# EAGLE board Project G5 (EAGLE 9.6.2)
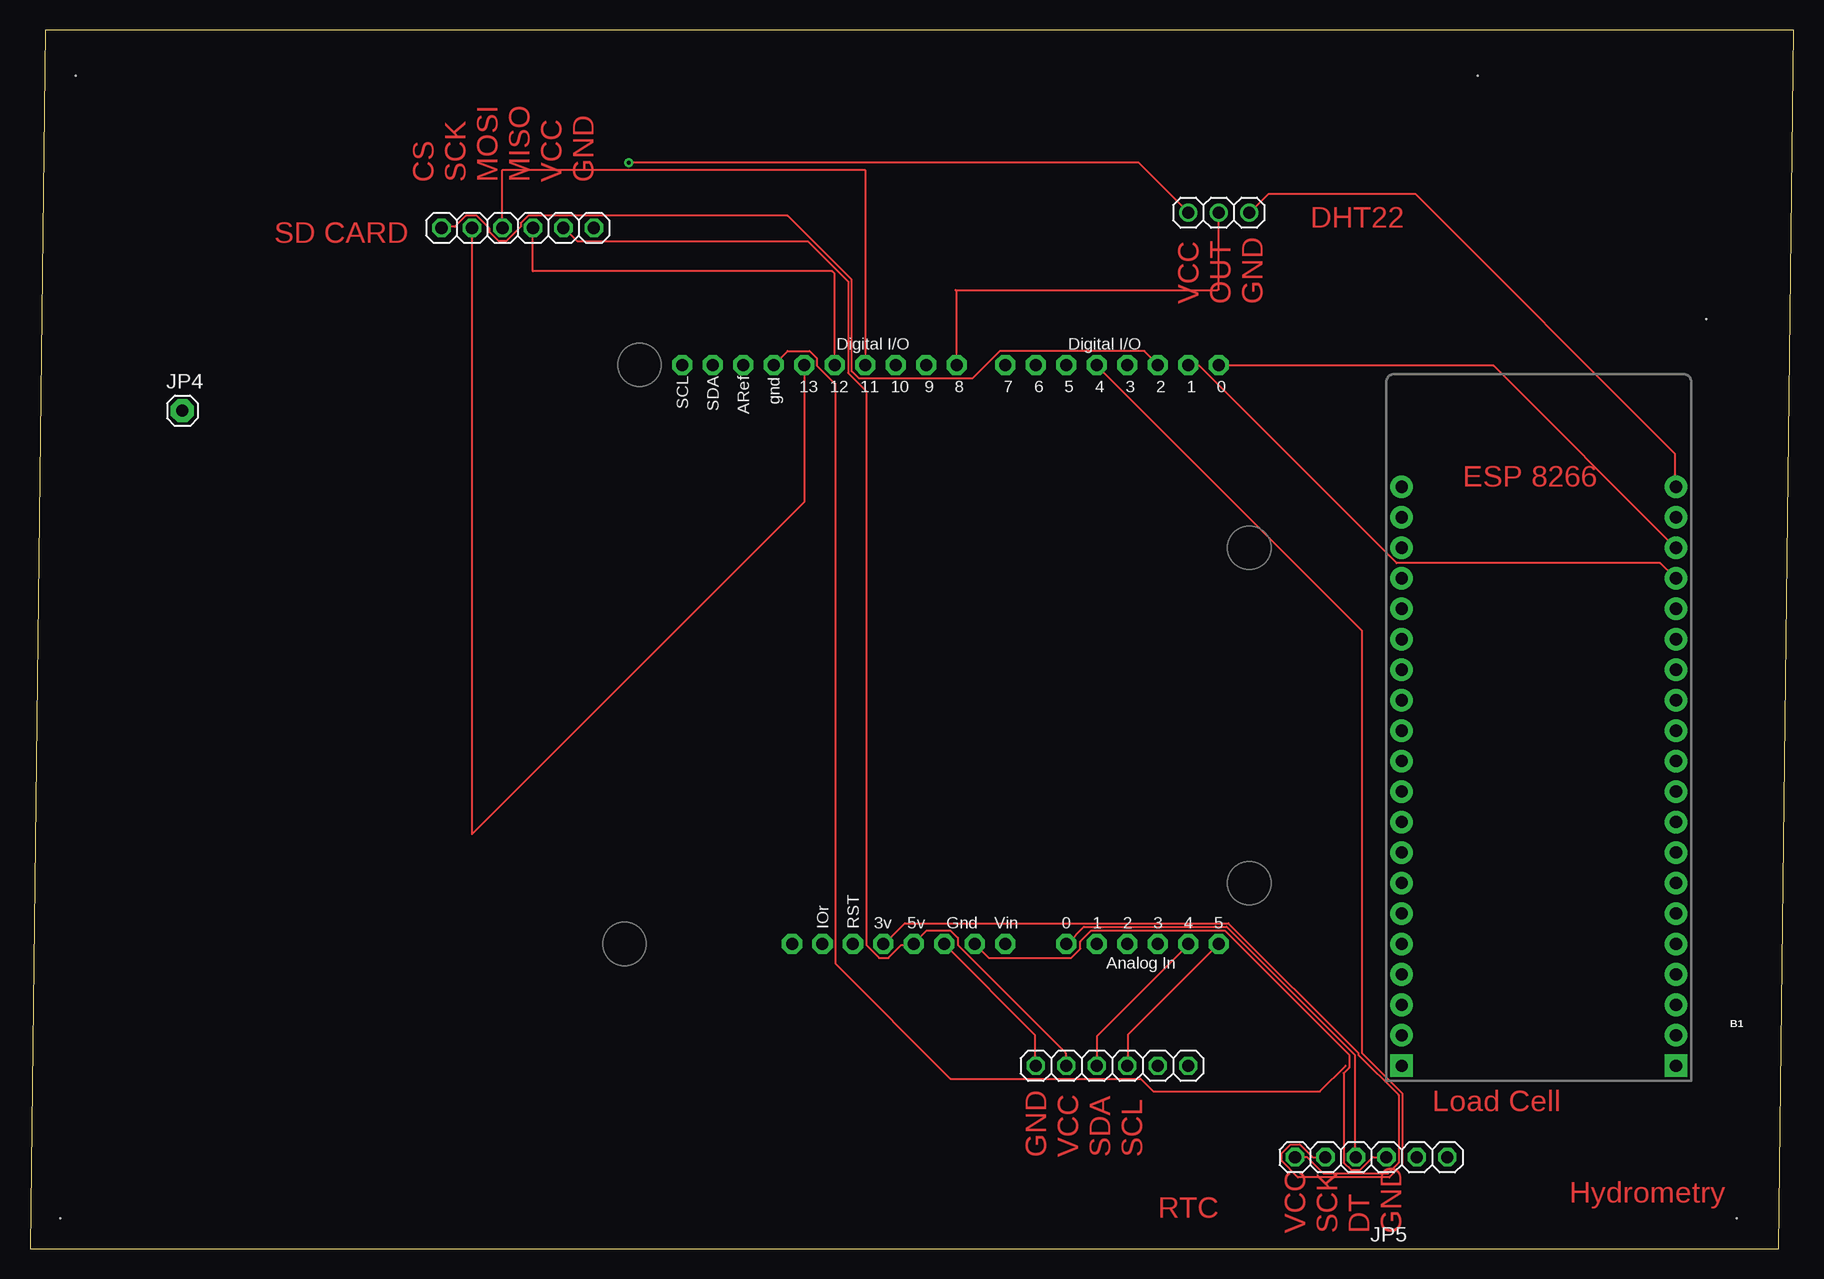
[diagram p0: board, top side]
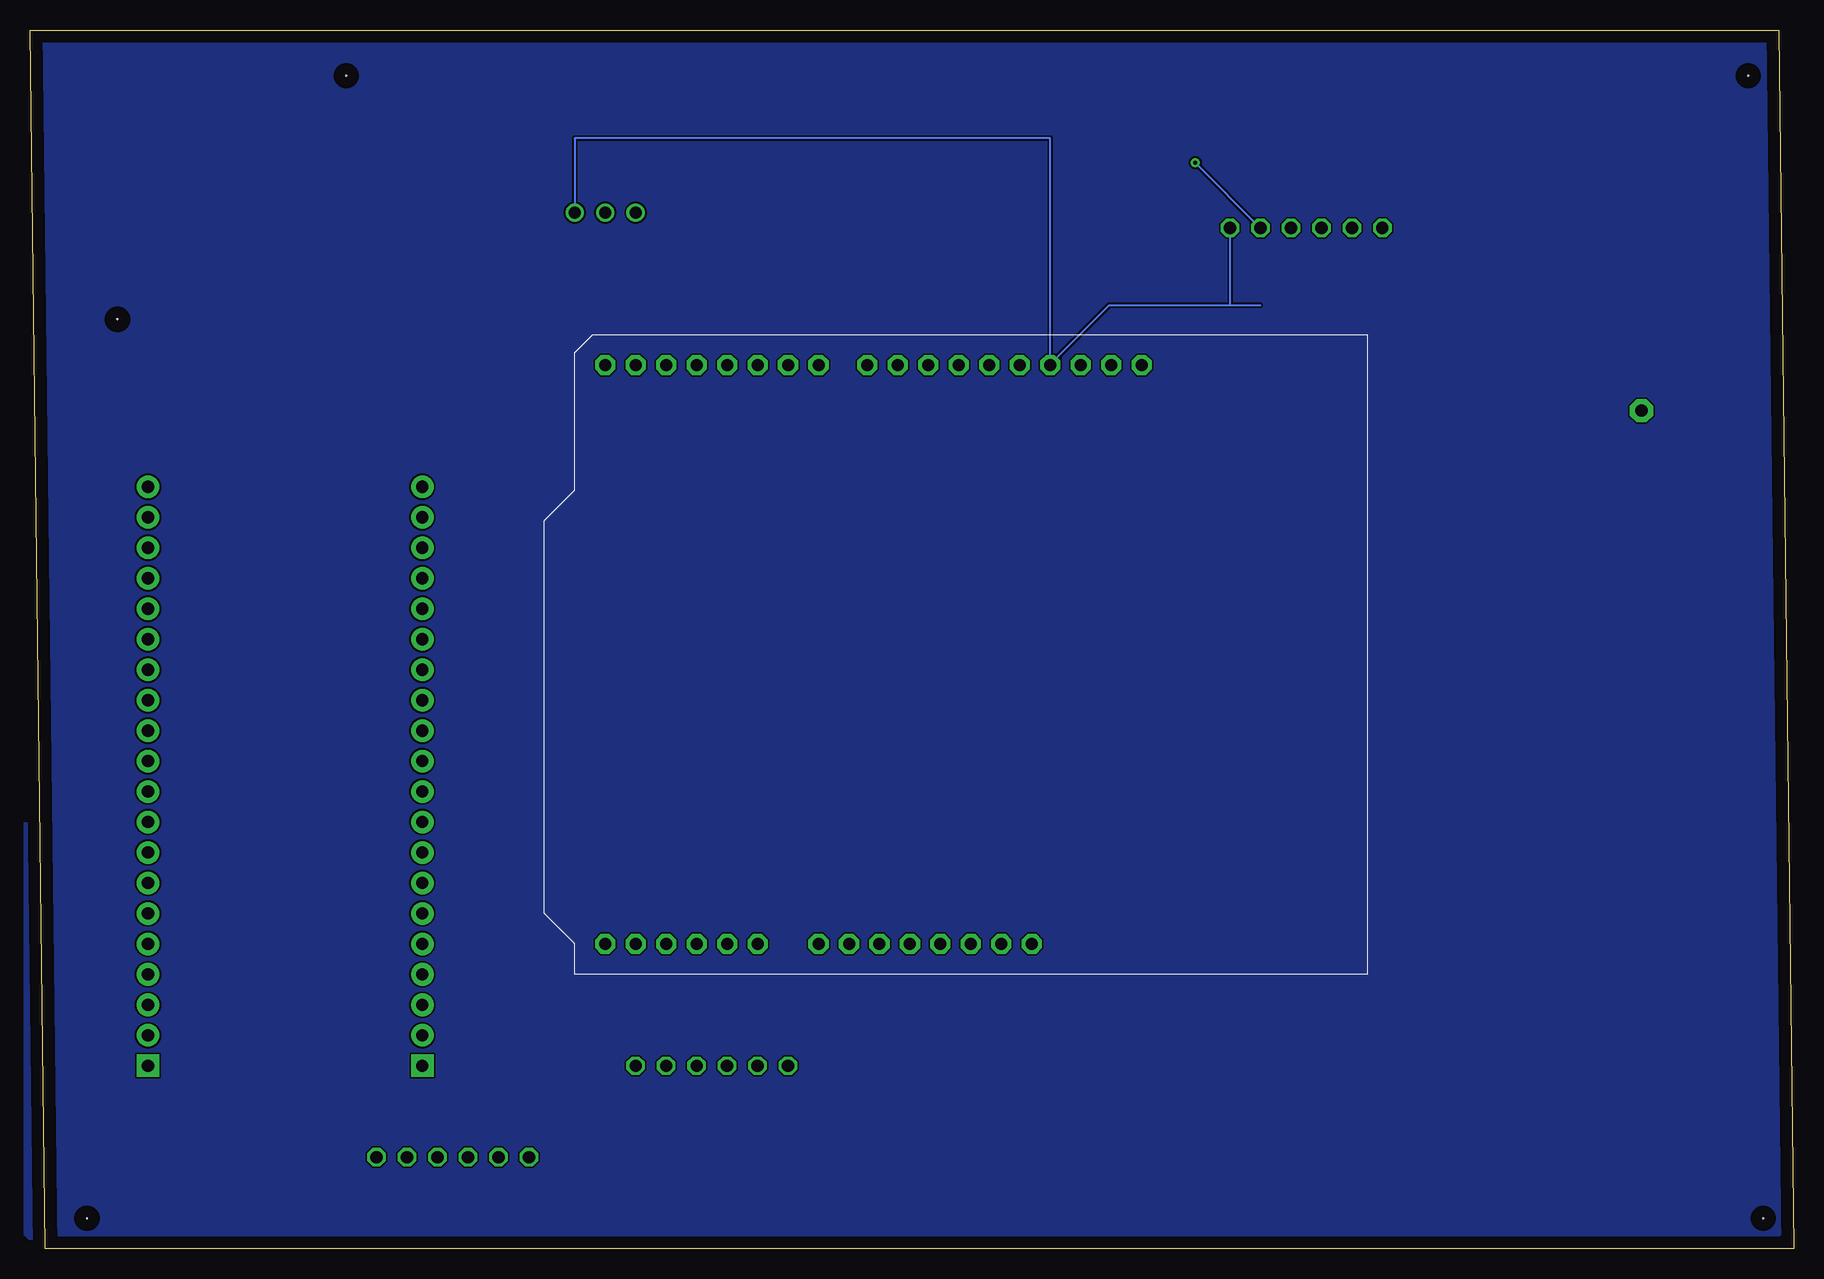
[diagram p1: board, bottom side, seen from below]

Size 146.99 x 101.59 mm. Coordinates in mm from the lower left corner, seen from the top.
Outline: 0,0 145.72,0 146.99,101.59 1.27,101.59 0,0
Copper layers (1*16): Top 0.035mm / dielectric 1.5mm / Bottom 0.035mm
Design rules "default": minimum track width 6mil, minimum drill 0.35mm, track to track 6mil, track to pad 6mil, pad to pad 6mil, via to via 6mil, smd to smd 6mil, copper to edge 40mil, drill to drill 6mil, minimum pad ring 10mil, minimum via ring 8mil, stop-mask expansion 4mil, vias tented up to drill 0mil, thermal gap 10mil
Holes 0.06 mm at 3.81,97.79 120.65,97.79 139.7,77.47 142.24,2.54 2.54,2.54

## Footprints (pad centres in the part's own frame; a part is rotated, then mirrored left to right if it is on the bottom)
ESP32_THING_NO_ANT = drill 1.016 pad 1.88 square: 1 1.27,1.27; 40 24.13,1.27 | drill 1.016 pad 1.88: 2 1.27,3.81; 3 1.27,6.35; 4 1.27,8.89; 5 1.27,11.43; 6 1.27,13.97; 7 1.27,16.51; 8 1.27,19.05; 9 1.27,21.59; 10 1.27,24.13; 11 1.27,26.67; 12 1.27,29.21; 13 1.27,31.75; 14 1.27,34.29; 15 1.27,36.83; 16 1.27,39.37; 17 1.27,41.91; 18 1.27,44.45; 19 1.27,46.99; 20 1.27,49.53; 21 24.13,49.53; 22 24.13,46.99; 23 24.13,44.45; 24 24.13,41.91; 25 24.13,39.37; 26 24.13,36.83; 27 24.13,34.29; 28 24.13,31.75; 29 24.13,29.21; 30 24.13,26.67; 31 24.13,24.13; 32 24.13,21.59; 33 24.13,19.05; 34 24.13,16.51; 35 24.13,13.97; 36 24.13,11.43; 37 24.13,8.89; 38 24.13,6.35; 39 24.13,3.81
1X03 = drill 1.016: 1 -2.54,0; 2 0,0; 3 2.54,0
1X06 = drill 1.016 octagon: 1 -6.35,0; 2 -3.81,0; 3 -1.27,0; 4 1.27,0; 5 3.81,0; 6 6.35,0
1X01 = drill 1.016 pad 1.93 octagon: 1 0,0
ARDUINOR3-BPLACE = drill 1 pad 1.676 octagon: 3V 35.56,2.54; 5V 38.1,2.54; A0 50.8,2.54; A1 53.34,2.54; A2 55.88,2.54; A3 58.42,2.54; A4 60.96,2.54; A5 63.5,2.54; AREF 23.876,50.8; D0 63.5,50.8; D1 60.96,50.8; D2 58.42,50.8; D3 55.88,50.8; D4 53.34,50.8; D5 50.8,50.8; D6 48.26,50.8; D7 45.72,50.8; D8 41.656,50.8; D9 39.116,50.8; D10 36.576,50.8; D11 34.036,50.8; D12 31.496,50.8; D13 28.956,50.8; GND 26.416,50.8; GND1 43.18,2.54; GND2 40.64,2.54; IOREF 30.48,2.54; RESERVED 27.94,2.54; RESET 33.02,2.54; SCL 18.796,50.8; SDA 21.336,50.8; VIN 45.72,2.54

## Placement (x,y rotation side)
B1  ESP32_THING_WO_ANT_KEEPOUT  [ESP32_THING_NO_ANT]  113.03,13.97 0 top
FRAME1  FRAME-LEDGER  [CREATIVE_COMMONS]  not placed on the board
JP1  [1X03]  99.06,86.36 0 top
JP2  [1X06]  40.64,85.09 0 top
JP3  [1X06]  90.17,15.24 0 top
JP4  [1X01]  12.7,69.85 0 top
JP5  [1X06]  111.76,7.62 0 top
U1  ARDUINOR3-BPLACE  [ARDUINOR3-BPLACE]  35.56,22.86 0 top

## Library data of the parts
B1 = SparkFun-Boards
FRAME1 = SparkFun-Aesthetics
JP1-JP5 U1 = adafruit

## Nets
N$1: JP5.2 U1.D4
N$2: B1.21 JP1.3 JP2.6 U1.GND
N$3: JP2.4 U1.D12
N$4: JP3.1 U1.GND2
N$5: JP2.1 U1.D2
N$6: JP3.3 U1.A4
N$7: B1.23 U1.D0
N$8: JP2.3 U1.D11
N$9: JP2.2 U1.D13
N$10: B1.1
N$11: B1.24 U1.D1
N$13: JP1.2 U1.D8
N$14: JP3.4 U1.A5
N$15: JP1.1 JP2.5 JP3.2 U1.5V
N$16: JP5.1 U1.3V
N$17: JP5.3 U1.A0
N$18: JP5.4 U1.GND1
VIN: U1.VIN

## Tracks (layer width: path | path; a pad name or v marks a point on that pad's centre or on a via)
GND
  pour Bottom: 1.27,101.6 120.65,101.6 143.51,78.74 143.51,1.27 1.27,1.27 1.27,100.33
  pour Bottom: 2.54,100.33 147.32,100.33 147.32,1.27 146.05,0 2.54,0 1.27,1.27 1.27,99.06
N$1
  Top 0.152: JP5.2 106.88,7.62 105.82,8.69 105.05,8.69 104.29,7.92 104.29,7.31 105.66,5.94 113.28,5.94 114.35,7.01 114.35,12.95 111,16.31 111,51.51 88.9,73.61 U1.D4
N$2
  Top 0.152: 109.63,15.24 107.49,13.11 93.62,13.11 92.56,14.17 76.71,14.17 67.11,23.77 67.11,72.09 65.58,73.61 65.58,74.22 64.97,74.83 63.14,74.83 U1.GND | B1.21 137.06,63.55 137.06,66.29 115.42,87.94 103.23,87.94 101.7,86.41 JP1.3
  Bottom 0.152: 46.99,78.64 57.05,78.64 61.92,73.76 U1.GND 61.98,92.56 101.6,92.56 JP1.3 | 46.99,78.64 44.45,78.64 | 46.99,78.64 JP2.6
N$3
  Top 0.152: JP2.4 41.91,81.48 66.85,81.48 67.06,81.28 U1.D12
N$4
  Top 0.152: JP3.1 83.72,15.24 83.72,17.83 76.25,25.3 U1.GND2
N$5
  Top 0.152: JP2.1 34.34,85.19 35.41,85.19 36.32,86.11 37.24,86.11 38.3,85.04 38.3,84.73 39.06,83.97 39.67,83.97 40.89,85.19 40.89,85.5 41.5,86.11 63.14,86.11 68.48,80.77 68.48,73.15 69.09,72.54 78.54,72.54 80.82,74.83 92.86,74.83 93.93,73.76 U1.D2
N$6
  Top 0.152: JP3.3 88.9,17.68 96.52,25.3 U1.A4
N$7
  Top 0.152: B1.23 121.97,73.61 99.11,73.61 U1.D0
N$8
  Top 0.152: JP2.3 39.37,89.92 69.6,89.92 U1.D11
N$9
  Top 0.152: JP2.2 36.83,34.54 64.52,62.23 U1.D13
N$11
  Top 0.152: U1.D1 96.52,73.61 97.43,73.61 113.89,57.15 135.84,57.15 137.06,55.93 B1.24
N$13
  Top 0.152: JP1.2 99.06,80.01 98.96,79.91 77.11,79.91 77.22,79.81 U1.D8
N$14
  Top 0.152: U1.A5 91.49,17.83 91.49,15.24 JP3.4
N$15  (via drill 0.35)
  Top 0.152: JP3.2 86.31,15.24 86.31,16.31 77.32,25.3 77.32,25.91 76.71,26.52 74.73,26.52 73.66,25.45 U1.5V 73.66,25.3 72.59,25.3 71.53,24.23 70.76,24.23 69.7,25.3 69.7,71.48 68.17,73 68.17,80.62 64.82,83.97 45.62,83.97 44.55,85.04 JP2.5 | v49.89,90.53 92.41,90.53 96.52,86.41 JP1.1
  Bottom 0.152: v49.89,90.53 JP2.5
N$16
  Top 0.152: JP5.1 106.43,7.62 107.8,6.25 113.13,6.25 114.05,7.16 114.05,12.8 110.69,16.15 110.69,16.31 99.87,27.13 72.9,27.13 71.22,25.45 U1.3V
N$17
  Top 0.152: JP5.3 110.39,7.62 110.39,16.15 99.72,26.82 87.83,26.82 86.46,25.45 U1.A0
N$18
  Top 0.152: JP5.4 111.91,7.62 110.85,6.55 110.08,6.55 109.47,7.16 109.47,14.63 109.93,15.09 109.93,16.15 99.57,26.52 88.44,26.52 87.53,25.6 87.53,24.99 86.77,24.23 79.91,24.23 U1.GND1

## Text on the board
Top: CS / SCK / MOSI / MISO / VCC / GND | DHT22 | SD CARD | VCC / OUT / GND | ESP 8266 | Load Cell | GND / VCC / SDA / SCL | Hydrometry | RTC | VCC / SCK / DT / GND

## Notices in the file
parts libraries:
SparkFun-Aesthetics: Licensing: Creative Commons ShareAlike 4.0 International - https://creativecommons.org/licenses/by-sa/4.0
SparkFun-Aesthetics: Released under the Creative Commons Attribution Share-Alike 4.0 License
SparkFun-Aesthetics: https://creativecommons.org/licenses/by-sa/4.0
